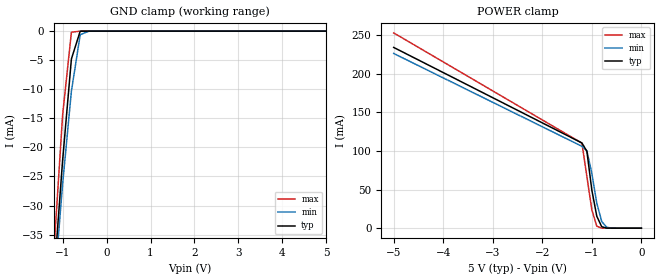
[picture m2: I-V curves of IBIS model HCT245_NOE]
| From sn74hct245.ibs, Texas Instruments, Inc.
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|   Model HCT245_NOE
[Model]   HCT245_NOE
Model_type  Input
Polarity   Inverting
Vinl = 0.8
Vinh = 2.0
| variable   typ   min   max
C_comp   3.0pf   NA   10pf
[Temperature Range]   25   85   -40
[Voltage Range]   5.0   4.5   5.5
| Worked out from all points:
|   GND clamp passes 1 mA (typ) near -0.64 V on its own axis
|   POWER clamp passes 1 mA (typ) near -0.75 V on its own axis
[GND Clamp]
|   Voltage   I(typ)   I(min)   I(max)
-5V       -578.5mA   -523.7mA   -635.1mA
-1.2V     -42.62mA   -44.98mA   -38.09mA
-1V       -22.25mA   -26.31mA   -14.44mA
-800mV    -4.791mA   -10.35mA   -193uA
-600mV    -22.16uA   -617.1uA   -2.711uA
-400mV    -9.918nA   -1.85uA    -2.522uA
5V        72.38pA    5.803uA    860.1nA
[POWER Clamp]
|   Voltage   I(typ)   I(min)   I(max)
-5V       233.8mA    226mA      252.6mA
-1.2V     110.2mA    105.9mA    110mA
-1.1V     99.53mA    100mA      66.88mA
-1V       49.32mA    71.06mA    23.77mA
-900mV    15.45mA    32.33mA    2.492mA
-800mV    1.779mA    8.583mA    49.28uA
-700mV    96uA       1.128mA    2.003uA
-600mV    2.976uA    100.3uA    1.529uA
0V        523.8pA    326.4pA    113nA
